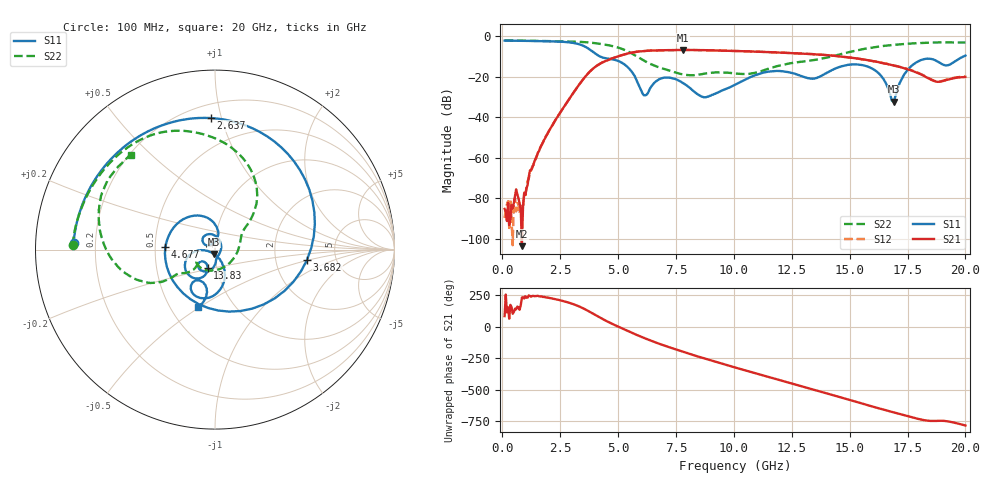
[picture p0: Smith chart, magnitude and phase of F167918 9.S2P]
!  2-Port S-parameters saved by WinCal
! VAR MeasName=S-Parameters (CALIBRATED_DATA) read from VNA (N5242A)
! VAR MeasDate=2016-11-22 10:25:16
! VAR NAME=F167918 9
! VAR FILENAME=F167918 9.S2P
! VAR DATE=2016-11-22 10:25:16
! VAR PHYS_PORTS=1,2
# Hz S DB R 50
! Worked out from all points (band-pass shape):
!   401 points, 100 MHz to 20 GHz, reference 50 ohm
!   highest |S21| = -6.70 dB at 7.811 GHz (marker M1); lowest = -103.7 dB at 846.2 MHz (marker M2)
!   |S21| within 3 dB of the highest: 5.041 GHz to 14.42 GHz (9.382 GHz wide, 96.4 % of centre)
!   lowest |S11| = -32.3 dB at 16.92 GHz (marker M3), VSWR 1.05, Z = 49.5 - j2.37 ohm
!   |S11| at or under -10 dB: 4.235 GHz to 19.9 GHz (15.66 GHz wide, 130 % of centre)
!   |S22| runs from -19.2 to -2.0 dB; largest |S21 - S12| = 0.0038
!   S11 on the Smith chart (normalised r, x): 100 MHz: 0.12, +0.02; 2.637 GHz: 0.29, +0.93; 3.682 GHz: 3.04, -0.49; 4.677 GHz: 0.57, +0.02; 13.83 GHz: 0.90, -0.19; 20 GHz: 0.68, -0.49
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1e8  -2.07 177.3  -85.27 82.1  -89.80 167.4  -2.00 178.3
8.4625e8  -2.18 157.3  -103.70 -131.8  -82.98 144.4  -2.13 166.6
1.64225e9  -2.32 133.7  -54.79 -122.7  -55.09 -122.8  -2.25 154.2
2.63725e9  -2.69 91.8  -35.28 -159.1  -35.26 -159.3  -2.43 136.8
3.43325e9  -4.33 26.8  -22.05 149.1  -22.08 149.1  -2.73 119.3
3.682e9  -5.76 -6.5  -18.59 125.8  -18.59 125.9  -2.94 112.9
4.08e9  -9.01 -77.1  -14.52 84.3  -14.47 84.2  -3.45 101.9
4.677e9  -11.15 177.4  -11.15 27.2  -11.12 26.8  -4.57 83.8
5.473e9  -15.86 96.1  -8.31 -39.2  -8.32 -39.6  -7.70 55.6
6.11975e9  -29.14 111.3  -7.20 -90.0  -7.21 -90.3  -11.95 39.6
6.7665e9  -21.24 143.6  -6.87 -135.4  -6.88 -135.6  -15.29 29.9
7.81125e9  -23.05 80.8  -6.70 160.1  -6.71 160.1  -18.84 -26.2
8.70675e9  -30.12 -16.1  -6.79 108.7  -6.80 108.7  -18.46 -100.2
1.005e10  -23.90 -85.4  -7.18 36.5  -7.20 36.7  -18.34 -148.8
1.19405e10  -17.08 -127.1  -8.02 -60.7  -7.98 -60.7  -14.48 -139.1
1.338325e10  -20.93 -126.9  -8.76 -134.7  -8.74 -134.4  -11.81 -147.2
1.3831e10  -19.13 -111.4  -9.12 -158.0  -9.07 -157.8  -10.91 -147.2
1.567175e10  -14.50 -153.1  -11.50 104.6  -11.52 104.7  -6.09 -162.7
1.67165e10  -27.68 -170.1  -13.84 51.0  -13.86 51.5  -4.41 -179.3
1.69155e10  -32.28 -100.6  -14.41 41.4  -14.32 41.6  -4.17 177.4
1.786075e10  -12.97 -82.7  -17.68 -5.4  -17.53 -4.8  -3.36 162.7
2e10  -9.47 -106.4  -20.04 -61.5  -19.83 -61.7  -3.02 131.8
